[IBIS ver]   4.1
[File name]   sprm642a.ibs
[File Rev]   1.0
[Notes]
   IO cell model for C2000
[Date]   Nov 21, 2013
[Source]   File originated at Texas Instruments
[Copyright]   (c) 2012, Texas Instruments Inc.
[Component]   f771553xptp
[Manufacturer] Texas Instruments
[Package]
| Variable   Typ   Min   Max
R_pkg   0.164   0.00678   0.207
L_pkg   7.99E-09   6.94E-09   9.66E-09
C_pkg   2.73E-12   2.18E-12   3.96E-12
[Pin] signal_name   model_name   R_pin   L_pin   C_pin
1   GPIO10   BCF183350CSHYPBFZ   2.07E-01   9.66E-09   2.25E-12
2   GPIO11   BCF183350CSHYPBFZ   2.03E-01   9.34E-09   3.02E-12
3   VDDSFL1833   NC   1.98E-01   9.27E-09   3.01E-12
4   GPIO12   BCF183350CSHYPBFZ   1.92E-01   8.96E-09   2.97E-12
5   GPIO13   BCF183350CSHYPBFZ   1.90E-01   8.86E-09   2.93E-12
6   GPIO14   BCF183350CSHYPBFZ   1.85E-01   8.70E-09   2.89E-12
7   GPIO15   BCF183350CSHYPBFZ   1.82E-01   8.48E-09   2.84E-12
8   GPIO16   BCF183350CSHYPBFZ   1.79E-01   8.37E-09   2.81E-12
9   GPIO17   BCF183350CSHYPBFZ   1.76E-01   8.17E-09   2.76E-12
10   GPIO18   BCF183350CSHYPBFZ   1.74E-01   8.07E-09   2.70E-12
11   VDDSFL1833   NC   1.73E-01   7.90E-09   2.65E-12
12   GPIO19   BCF183350CSHYPBFZ   1.72E-01   7.79E-09   2.62E-12
13   GPIO20   BCF183350CSHYPBFZ   1.71E-01   7.75E-09   2.59E-12
14   GPIO21   BCF183350CSHYPBFZ   1.71E-01   7.59E-09   2.55E-12
15   VDDSFL   NC   1.72E-01   7.56E-09   2.52E-12
16   VDD   NC   1.72E-01   7.53E-09   2.48E-12
17   VPP   NC   9.16E-02   7.04E-09   2.94E-12
18   GPIO8   BCF3350CSHYPBFZ   1.74E-01   7.41E-09   2.43E-12
19   GPIO9   BCF3350CSHYPBFZ   1.74E-01   7.27E-09   2.40E-12
20   VDDSFL   NC   1.75E-01   7.31E-09   2.44E-12
21   VDD   NC   1.75E-01   7.17E-09   3.56E-12
22   GPIO22   BCF3350CSHYPBFZ   1.77E-01   7.39E-09   2.42E-12
23   GPIO23   BCF3350CSHYPBFZ   1.76E-01   7.29E-09   2.44E-12
24   GPIO24   BCF3350CSHYPBFZ   1.76E-01   7.24E-09   2.41E-12
25   GPIO25   BCF3350CSHYPBFZ   1.75E-01   7.32E-09   2.40E-12
26   VDDSFL   NC   1.75E-01   7.31E-09   2.39E-12
27   GPIO26   BCF3350CSHYPBFZ   1.75E-01   7.38E-09   2.41E-12
28   GPIO27   BCF3350CSHYPBFZ   1.76E-01   7.44E-09   2.40E-12
29   ADCINC4   NC   1.76E-01   7.49E-09   2.43E-12
30   ADCINC3   NC   1.75E-01   7.51E-09   2.50E-12
31   ADCINC2   NC   1.74E-01   7.60E-09   2.55E-12
32   ADCINC1   NC   1.74E-01   7.67E-09   2.60E-12
33   ADCINC0   NC   1.74E-01   7.80E-09   2.65E-12
34   VSSA   NC   1.75E-01   7.84E-09   2.71E-12
35   VREFHI3   NC   9.36E-02   7.64E-09   3.39E-12
36   VDDA   NC   9.37E-02   7.69E-09   3.48E-12
37   VREFHI1   NC   9.43E-02   7.85E-09   3.53E-12
38   ADCINA5   NC   9.49E-02   7.97E-09   3.52E-12
39   ADCINA4   NC   1.80E-01   8.46E-09   2.92E-12
40   ADCINA3   NC   1.82E-01   8.72E-09   2.95E-12
41   ADCINA2   NC   1.86E-01   8.78E-09   2.98E-12
42   ADCINA1   NC   1.90E-01   8.94E-09   3.01E-12
43   ADCINA0   NC   1.95E-01   9.19E-09   3.03E-12
44   ADCINCAL0   NC   2.00E-01   9.52E-09   2.27E-12
45   ADCINCAL1   NC   1.72E-01   9.30E-09   2.25E-12
46   ADCINB0   NC   1.66E-01   9.01E-09   3.05E-12
47   ADCINB1   NC   1.63E-01   8.95E-09   3.04E-12
48   ADCINB2   NC   1.59E-01   8.56E-09   3.00E-12
49   ADCINB3   NC   1.56E-01   8.52E-09   2.95E-12
50   ADCINB4   NC   1.54E-01   8.36E-09   2.90E-12
51   ADCINB5   NC   1.52E-01   8.19E-09   2.84E-12
52   VSSA   NC   8.44E-02   8.01E-09   3.36E-12
53   VREFHI2   NC   8.38E-02   7.79E-09   3.39E-12
54   VDDA   NC   8.35E-02   7.72E-09   3.36E-12
55   VREFHI4   NC   8.31E-02   7.60E-09   3.30E-12
56   ADCIND0   NC   1.53E-01   7.61E-09   2.70E-12
57   ADCIND1   NC   1.52E-01   7.63E-09   2.64E-12
58   ADCIND2   NC   1.52E-01   7.52E-09   2.58E-12
59   ADCIND3   NC   1.52E-01   7.43E-09   2.53E-12
60   ADCIND4   NC   1.53E-01   7.32E-09   2.46E-12
61   VDD   NC   1.58E-01   7.52E-09   2.40E-12
62   VDDSFL   NC   1.57E-01   7.34E-09   2.42E-12
63   GPIO30   BCF3355DSHYPBFZ   1.57E-01   7.16E-09   2.42E-12
64   GPIO28   BCF3385DSHYPBFZ   1.56E-01   7.30E-09   2.41E-12
65   GPIO29   BCF3385DSHYPBFZ   1.55E-01   7.15E-09   2.38E-12
66   GPIO31   BCF3385DSHYPBFZ   1.55E-01   7.23E-09   2.29E-12
67   GPIO32   BCF3385DSHYPBFZ   1.57E-01   7.26E-09   2.32E-12
68   VDDSFL   NC   1.56E-01   7.23E-09   2.41E-12
69   GPIO33   BCF3385DSHYPBFZ   1.53E-01   7.13E-09   2.43E-12
70   GPIO34   BCF3385DSHYPBFZ   1.52E-01   7.18E-09   2.45E-12
71   GPIO35   BCF3385DSHYPBFZ   1.50E-01   7.12E-09   2.45E-12
72   VDD3VFL   NC   7.87E-02   6.94E-09   2.89E-12
73   FLT1   NC   1.46E-01   7.32E-09   2.46E-12
74   FLT2   NC   1.45E-01   7.25E-09   2.48E-12
75   VDDSFL   NC   1.48E-01   7.47E-09   2.58E-12
76   VDD   NC   1.47E-01   7.42E-09   3.55E-12
77   TDI   BCF3335DSHYPBFZ   1.47E-01   7.64E-09   2.64E-12
78   TDO   BCF3335DSHYPBFZ   1.46E-01   7.81E-09   2.67E-12
79   TRSTn   BCF3335CSHYPBFZ   1.46E-01   7.84E-09   2.69E-12
80   TMS   IQ0442FS_40P60P_3X2   1.46E-01   8.01E-09   2.71E-12
81   TCK   IQ0442FS_40P60P_3X2   1.46E-01   8.05E-09   2.75E-12
82   VDDSFL   NC   1.46E-01   8.21E-09   2.79E-12
83   GPIO36   BCF3385DSHYPBFZ   1.46E-01   8.25E-09   2.85E-12
84   GPIO37   BCF3385DSHYPBFZ   1.47E-01   8.41E-09   2.91E-12
85   GPIO38   BCF3385DSHYPBFZ   1.49E-01   8.54E-09   2.96E-12
86   GPIO39   BCF3385DSHYPBFZ   1.52E-01   8.80E-09   2.98E-12
87   GPIO40   BCF3385DSHYPBFZ   1.53E-01   8.92E-09   2.99E-12
88   VDDSFL   NC   1.55E-01   8.99E-09   2.23E-12
89   GPIO41   BCF3385DSHYPBFZ   1.77E-01   9.22E-09   2.18E-12
90   GPIO48   BCF3385DSHYPBFZ   1.73E-01   9.12E-09   2.92E-12
91   VDDSFL   NC   1.69E-01   8.83E-09   2.91E-12
92   ERRORSTS   BCF3350BSHYPBFZ   1.66E-01   8.63E-09   2.87E-12
93   GPIO49   BCF3385DSHYPBFZ   1.63E-01   8.50E-09   2.83E-12
94   GPIO50   BCF3385DSHYPBFZ   1.59E-01   8.25E-09   2.80E-12
95   GPIO51   BCF3385DSHYPBFZ   1.56E-01   8.24E-09   2.75E-12
96   GPIO52   BCF3385DSHYPBFZ   1.52E-01   7.95E-09   2.71E-12
97   GPIO53   BCF3385DSHYPBFZ   1.50E-01   7.79E-09   2.66E-12
98   GPIO54   BCF3385DSHYPBFZ   1.48E-01   7.68E-09   2.61E-12
99   VDDSFL   NC   1.47E-01   7.64E-09   2.57E-12
100   GPIO55   BCF3385DSHYPBFZ   1.47E-01   7.48E-09   2.53E-12
101   GPIO56   BCF3385DSHYPBFZ   1.47E-01   7.31E-09   2.50E-12
102   GPIO57   BCF3385DSHYPBFZ   1.48E-01   7.20E-09   2.46E-12
103   GPIO58   BCF3385DSHYPBFZ   1.48E-01   7.19E-09   2.42E-12
104   GPIO59   BCF3335DSHYPBFZ   1.50E-01   7.14E-09   2.37E-12
105   GPIO60   BCF3385DSHYPBFZ   1.51E-01   6.96E-09   2.34E-12
106   VDDSFL   NC   1.51E-01   7.04E-09   2.33E-12
107   GPIO61   BCF3335DSHYPBFZ   1.52E-01   7.01E-09   2.33E-12
108   GPIO62   BCF3385DSHYPBFZ   1.54E-01   7.06E-09   2.35E-12
109   GPIO63   BCF3385DSHYPBFZ   1.56E-01   7.10E-09   2.35E-12
110   GPIO64   BCF3335DSHYPBFZ   1.59E-01   7.06E-09   2.35E-12
111   GPIO65   BCF3385DSHYPBFZ   1.62E-01   7.29E-09   2.33E-12
112   GPIO66   BCF3335DSHYPBFZ   1.63E-01   7.14E-09   2.38E-12
113   GPIO44   BCF3385DSHYPBFZ   1.65E-01   7.14E-09   2.41E-12
114   VDDSFL   NC   1.66E-01   7.23E-09   2.40E-12
115   GPIO45   BCF3385DSHYPBFZ   1.68E-01   7.30E-09   2.40E-12
116   VDDSFL   NC   1.62E-01   7.25E-09   2.45E-12
117   VDD   NC   1.60E-01   7.30E-09   3.56E-12
118   GPIO133   BCF3350BSHYPBFZ   1.63E-01   7.45E-09   2.52E-12
119   VREGENZ   IQ0440FS_3X2_7LM   1.66E-01   7.60E-09   2.54E-12
120   VDDSFL1   NC   1.69E-01   7.79E-09   2.57E-12
121   X2   NC   1.71E-01   7.78E-09   2.60E-12
122   VSS.OSC   NC   1.74E-01   8.15E-09   2.64E-12
123   X1   NC   1.79E-01   8.15E-09   2.66E-12
124   XRSn   BQ0491FS_3X2_7LM   1.74E-01   8.11E-09   2.71E-12
125   VDDSFL1   NC   1.76E-01   8.29E-09   2.81E-12
126   VDD   NC   6.78E-02   7.88E-09   3.96E-12
127   VDDSFL2   NC   9.38E-02   8.22E-09   3.38E-12
128   GPIO46   GPIOUSBV4_NFS_7LM   1.73E-01   8.62E-09   2.86E-12
129   GPIO47   GPIOUSBV4_NFS_7LM   1.78E-01   8.91E-09   2.91E-12
130   GPIO42   GPIOUSBV4_NFS_7LM   1.83E-01   9.10E-09   2.93E-12
131   GPIO43   GPIOUSBV4_NFS_7LM   1.86E-01   9.13E-09   2.93E-12
132   GPIO67   BCF3385DSHYPBFZ   1.91E-01   9.18E-09   2.19E-12
133   GPIO68   BCF3385DSHYPBFZ   1.84E-01   9.45E-09   2.29E-12
134   GPIO69   BCF3385DSHYPBFZ   1.83E-01   9.11E-09   3.06E-12
135   GPIO70   BCF3335DSHYPBFZ   1.81E-01   9.11E-09   3.04E-12
136   GPIO71   BCF3385DSHYPBFZ   1.80E-01   9.03E-09   3.00E-12
137   VDD   NC   1.79E-01   8.78E-09   2.97E-12
138   VDDSFL   NC   1.77E-01   8.85E-09   2.95E-12
139   GPIO72   BCF3335DSHYPBFZ   1.77E-01   8.55E-09   2.92E-12
140   GPIO73   BCF3385DSHYPBFZ   1.75E-01   8.52E-09   2.88E-12
141   GPIO74   BCF3385DSHYPBFZ   1.74E-01   8.26E-09   2.85E-12
142   GPIO75   BCF3385DSHYPBFZ   1.74E-01   8.18E-09   2.81E-12
143   GPIO76   BCF3385DSHYPBFZ   1.74E-01   8.08E-09   2.77E-12
144   GPIO77   BCF3385DSHYPBFZ   1.74E-01   7.96E-09   2.73E-12
145   GPIO78   BCF3385DSHYPBFZ   1.75E-01   7.90E-09   2.70E-12
146   GPIO79   BCF3385DSHYPBFZ   1.76E-01   7.78E-09   2.66E-12
147   VDDSFL   NC   1.77E-01   7.79E-09   2.63E-12
148   GPIO80   BCF3385DSHYPBFZ   1.78E-01   7.77E-09   2.60E-12
149   GPIO81   BCF3385DSHYPBFZ   1.80E-01   7.75E-09   2.58E-12
150   GPIO82   BCF3385DSHYPBFZ   1.82E-01   7.70E-09   2.55E-12
151   GPIO83   BCF3385DSHYPBFZ   1.85E-01   7.76E-09   2.50E-12
152   VDDSFL   NC   1.81E-01   7.56E-09   2.52E-12
153   VDD   NC   1.82E-01   7.60E-09   3.64E-12
154   GPIO84   BCF3385DSHYPBFZ   1.81E-01   7.62E-09   2.43E-12
155   GPIO85   BCF3385DSHYPBFZ   1.83E-01   7.67E-09   2.46E-12
156   GPIO86   BCF3385DSHYPBFZ   1.83E-01   7.54E-09   2.51E-12
157   GPIO87   BCF3385DSHYPBFZ   1.84E-01   7.64E-09   2.49E-12
158   VDD   NC   1.78E-01   7.56E-09   3.64E-12
159   VDDSFL   NC   1.78E-01   7.62E-09   2.55E-12
160   GPIO0   GPIORETV2_NFS   1.74E-01   7.67E-09   2.55E-12
161   GPIO1   GPIORETV2_NFS   1.74E-01   7.68E-09   2.60E-12
162   GPIO2   GPIORETV2_NFS   1.74E-01   7.66E-09   2.63E-12
163   GPIO3   GPIORETV2_NFS   1.75E-01   7.78E-09   2.67E-12
164   GPIO4   GPIORETV2_NFS   1.76E-01   7.91E-09   2.71E-12
165   GPIO5   GPIORETV2_NFS   1.78E-01   8.06E-09   2.75E-12
166   GPIO6   GPIORETV2_NFS   1.79E-01   8.20E-09   2.78E-12
167   GPIO7   GPIORETV2_NFS   1.82E-01   8.28E-09   2.81E-12
168   VDDSFL   NC   1.84E-01   8.73E-09   2.89E-12
169   VDD   NC   9.91E-02   8.26E-09   3.52E-12
170   GPIO88   BCF3385DSHYPBFZ   1.87E-01   8.74E-09   2.98E-12
171   GPIO89   BCF3385DSHYPBFZ   1.90E-01   8.89E-09   3.03E-12
172   GPIO90   BCF3385DSHYPBFZ   1.94E-01   9.02E-09   3.07E-12
173   GPIO91   BCF3385DSHYPBFZ   1.98E-01   9.32E-09   3.08E-12
174   GPIO92   BCF3385DSHYPBFZ   2.00E-01   9.37E-09   3.09E-12
175   GPIO93   BCF3385DSHYPBFZ   2.02E-01   9.49E-09   3.10E-12
176   GPIO94   BCF3385DSHYPBFZ   2.01E-01   9.61E-09   2.31E-12
| End of package information
|   Component BCF3335DSHYPBFZ
[Component]   BCF3335DSHYPBFZ
[Manufacturer]   Texas Instruments
[Package]
|  variable   typ   min   max
R_pkg   0   0   0
L_pkg   0   0   0
C_pkg   0   0   0
[Pin]   signal_name   model_name   R_pin   L_pin   C_pin
VSS   VSS   GND
VDDS   VDDS   POWER
PAD   PAD   BCF3335DSHYPBFZ
[Model Selector] BCF3335DSHYPBFZ
BCF3335D_WK_PU_ON  Cell operated at 3.3(nom)
|BCF3335D_WK_PU_ON; WEAK_PULLUP_ON
BCF3335D_DRIVER_MODE  Cell operated at 3.3(nom)
|BCF3335D_DRIVER_MODE
BCF3335D_WK_PD_ON  Cell operated at 3.3(nom)
|   Component BCF3385DSHYPBFZ
[Component]   BCF3385DSHYPBFZ
[Manufacturer]   Texas Instruments
[Package]
|  variable   typ   min   max
R_pkg   0   0   0
L_pkg   0   0   0
C_pkg   0   0   0
[Pin]   signal_name   model_name   R_pin   L_pin   C_pin
VSS   VSS   GND
VDDS   VDDS   POWER
PAD   PAD   BCF3385DSHYPBFZ
[Model Selector] BCF3385DSHYPBFZ
BCF3385D_WK_PU_ON  Cell operated at 3.3(nom)
|BCF3385D_WK_PU_ON; WEAK_PULLUP_ON
BCF3385D_DRIVER_MODE  Cell operated at 3.3(nom)
|BCF3385D_DRIVER_MODE
BCF3385D_WK_PD_ON  Cell operated at 3.3(nom)
|   Component BCF183350CSHYPBFZ
[Component]   BCF183350CSHYPBFZ
[Manufacturer]   Texas Instruments
[Package]
|  variable   typ   min   max
R_pkg   0   0   0
L_pkg   0   0   0
C_pkg   0   0   0
[Pin]   signal_name   model_name   R_pin   L_pin   C_pin
VSS   VSS   GND
VDDS   VDDS   POWER
PAD   PAD   BCF183350CSHYPBFZ
[Model Selector] BCF183350CSHYPBFZ
BCF183350C_WK_PU_ON_3P3V  Cell operated at 3.3(nom)
|BCF183350C_WK_PU_ON_3P3V; WEAK_PULLUP_ON
BCF183350C_DRVR_MODE_3P3V  Cell operated at 3.3(nom)
|BCF183350C_DRVR_MODE_3P3V
BCF183350C_WK_PD_ON_3P3V  Cell operated at 3.3(nom)
|BCF183350C_WK_PD_ON_3P3V; WEAK_PULLDOWN_ON
BCF183350C_WK_PU_ON_1P8  Cell operated at 1.8(nom)
|BCF183350C_WK_PU_ON_1P8; WEAK_PULLUP_ON
BCF183350C_DRVR_MODE_1P8  Cell operated at 1.8(nom)
|BCF183350C_DRVR_MODE_1P8
BCF183350C_WK_PD_ON_1P8  Cell operated at 1.8(nom)
|   Component IQ0442FS_40P60P_3X2
[Component]   IQ0442FS_40P60P_3X2
[Manufacturer]   Texas Instruments
[Package]
|  variable   typ   min   max
R_pkg   0   0   0
L_pkg   0   0   0
C_pkg   0   0   0
[Pin]   signal_name   model_name   R_pin   L_pin   C_pin
VSS   VSS   GND
VDDS   VDDS   POWER
PAD   PAD   IQ0442FS_40P60P_3X2
[Model Selector] IQ0442FS_40P60P_3X2
S_40P60P_3X2_7LM_3P3  Cell operated at 3.3(nom)
|IQ0442FS_40P60P_3X2_3P3; PUPD_OFF
0P60P_3X2_7LM_PU_3P3  Cell operated at 3.3(nom)
|IQ0442FS_40P60P_3X2_PU_3P3; PULLUP_ON
0P60P_3X2_7LM_PD_3P3  Cell operated at 3.3(nom)
|   Component IQ0440FS_3X2_7LM
[Component]   IQ0440FS_3X2_7LM
[Manufacturer]   Texas Instruments
[Package]
|  variable   typ   min   max
R_pkg   0   0   0
L_pkg   0   0   0
C_pkg   0   0   0
[Pin]   signal_name   model_name   R_pin   L_pin   C_pin
VSS   VSS   GND
VDDS   VDDS   POWER
PAD   PAD   IQ0440FS_3X2_7LM
[Model Selector] IQ0440FS_3X2_7LM
440FS_3X2_7LM_PD_3P3  Cell operated at 3.3(nom)
|IQ0440FS_3X2_7LM_PD_3P3; PULLDOWN_ON
IQ0440FS_3X2_7LM_3P3  Cell operated at 3.3(nom)
|   Component BQ0491FS_3X2_7LM
[Component]   BQ0491FS_3X2_7LM
[Manufacturer]   Texas Instruments
[Package]
|  variable   typ   min   max
R_pkg   0   0   0
L_pkg   0   0   0
C_pkg   0   0   0
[Pin]   signal_name   model_name   R_pin   L_pin   C_pin
VSS   VSS   GND
VDDS   VDDS   POWER
PAD   PAD   BQ0491FS_3X2_7LM
[Model Selector] BQ0491FS_3X2_7LM
491FS_3X2_7LM_PU_3P3  Cell operated at 3.3(nom)
|BQ0491FS_3X2_7LM_PU_3P3; PULLUP_ON
491FS_3X2_7LM_PZ_3P3  Cell operated at 3.3(nom)
|   Component GPIORETV2_NFS
[Component]   GPIORETV2_NFS
[Manufacturer]   Texas Instruments
[Package]
|  variable   typ   min   max
R_pkg   0   0   0
L_pkg   0   0   0
C_pkg   0   0   0
[Pin]   signal_name   model_name   R_pin   L_pin   C_pin
VSS   VSS   GND
VDDS   VDDS   POWER
PAD   PAD   GPIORETV2_NFS
[Model Selector] GPIORETV2_NFS
GPIORET_WK_PD_ON_3P3  Cell operated at 3.3(nom)
|GPIORET_WK_PD_ON_3P3; WEAK_PULLDOWN_ON
RET_8MA_OPEN_DRAIN  Cell operated at 3.3(nom)
|RET_8MA_OPEN_DRAIN; 8MA_OPEN_DRAIN_SLW
RET_DRVR_2MA_PUPDOFF  Cell operated at 3.3(nom)
|RET_DRVR_2MA_PUPDOFF
RET_4MA_OPEN_DRAIN  Cell operated at 3.3(nom)
|RET_4MA_OPEN_DRAIN; 4MA_OPEN_DRAIN
GPIORET_WK_PU_ON_3P3  Cell operated at 3.3(nom)
|GPIORET_WK_PU_ON_3P3; WEAK_PULLUP_ON
RET_2MA_OPEN_DRAIN  Cell operated at 3.3(nom)
|RET_2MA_OPEN_DRAIN; 2MA_OPEN_DRAIN
RET_DRVR_8MA_PUPDOFF  Cell operated at 3.3(nom)
|RET_DRVR_8MA_PUPDOFF
RET_DRVR_MODE_8MA_PUPDOFF_SLEW  Cell operated at 3.3(nom)
|RET_DRVR_MODE_8MA_PUPDOFF_SLEW
RET_DRVR_MODE_4MA_PUPDOFF  Cell operated at 3.3(nom)
|RET_DRVR_MODE_4MA_PUPDOFF
RET_8MA_OPEN_DRAIN_3P3  Cell operated at 3.3(nom)
|   Component BCF3335CSHYPBFZ
[Component]   BCF3335CSHYPBFZ
[Manufacturer]   Texas Instruments
[Package]
|  variable   typ   min   max
R_pkg   0   0   0
L_pkg   0   0   0
C_pkg   0   0   0
[Pin]   signal_name   model_name   R_pin   L_pin   C_pin
VSS   VSS   GND
VDDS   VDDS   POWER
PAD   PAD   BCF3335CSHYPBFZ
[Model Selector] BCF3335CSHYPBFZ
BCF3335C_WK_PU_ON_3P3  Cell operated at 3.3(nom)
|BCF3335C_WK_PU_ON_3P3; WEAK_PULLUP_ON
BCF3335C_DRIVER_MODE_3P3  Cell operated at 3.3(nom)
|BCF3335C_DRIVER_MODE_3P3
BCF3335C_WK_PD_ON_3P3  Cell operated at 3.3(nom)
|   Component BCF3350CSHYPBFZ
[Component]   BCF3350CSHYPBFZ
[Manufacturer]   Texas Instruments
[Package]
|  variable   typ   min   max
R_pkg   0   0   0
L_pkg   0   0   0
C_pkg   0   0   0
[Pin]   signal_name   model_name   R_pin   L_pin   C_pin
VSS   VSS   GND
VDDS   VDDS   POWER
PAD   PAD   BCF3350CSHYPBFZ
[Model Selector] BCF3350CSHYPBFZ
BCF3350C_WK_PU_ON_3P3  Cell operated at 3.3(nom)
|BCF3350C_WK_PU_ON_3P3; WEAK_PULLUP_ON
BCF3350C_DRIVER_MODE_3P3  Cell operated at 3.3(nom)
|BCF3350C_DRIVER_MODE_3P3
BCF3350C_WK_PD_ON_3P3  Cell operated at 3.3(nom)
|   Component BCF3350BSHYPBFZ
[Component]   BCF3350BSHYPBFZ
[Manufacturer]   Texas Instruments
[Package]
|  variable   typ   min   max
R_pkg   0   0   0
L_pkg   0   0   0
C_pkg   0   0   0
[Pin]   signal_name   model_name   R_pin   L_pin   C_pin
VSS   VSS   GND
VDDS   VDDS   POWER
PAD   PAD   BCF3350BSHYPBFZ
[Model Selector] BCF3350BSHYPBFZ
BCF3350B_WK_PU_ON_3P3  Cell operated at 3.3(nom)
|BCF3350B_WK_PU_ON_3P3; WEAK_PULLUP_ON
BCF3350B_DRIVER_MODE_3P3  Cell operated at 3.3(nom)
|BCF3350B_DRIVER_MODE_3P3
BCF3350B_WK_PD_ON_3P3  Cell operated at 3.3(nom)
|   Component GPIOUSBV4_NFS_7LM
[Component]   GPIOUSBV4_NFS_7LM
[Manufacturer]   Texas Instruments
[Package]
|  variable   typ   min   max
R_pkg   0   0   0
L_pkg   0   0   0
C_pkg   0   0   0
[Pin]   signal_name   model_name   R_pin   L_pin   C_pin
VSS   VSS   GND
VDDS   VDDS   POWER
PAD   PAD   GPIOUSBV4_NFS_7LM
[Model Selector] GPIOUSBV4_NFS_7LM
GPIOUSB_WK_PD_ON_3P3  Cell operated at 3.3(nom)
|GPIOUSB_WK_PD_ON_3P3; WEAK_PULLDOWN_ON
USB_8MA_OPEN_DRAIN_SLW  Cell operated at 3.3(nom)
|USB_8MA_OPEN_DRAIN_SLW; 8MA_OPEN_DRAIN_SLW
USB_DRVR_2MA_PUPDOFF  Cell operated at 3.3(nom)
|USB_DRVR_2MA_PUPDOFF
USB_4MA_OPEN_DRAIN  Cell operated at 3.3(nom)
|USB_4MA_OPEN_DRAIN; 4MA_OPEN_DRAIN
GPIOUSB_WK_PU_ON_3P3  Cell operated at 3.3(nom)
|GPIOUSB_WK_PU_ON_3P3; WEAK_PULLUP_ON
USB_2MA_OPEN_DRAIN  Cell operated at 3.3(nom)
|USB_2MA_OPEN_DRAIN; 2MA_OPEN_DRAIN
USB_DRVR_8MA_PUPDOFF  Cell operated at 3.3(nom)
|USB_DRVR_8MA_PUPDOFF
USB_DRVR_8MA_PUPDOFF_SLW  Cell operated at 3.3(nom)
|USB_DRVR_8MA_PUPDOFF_SLW
USB_DRVR_4MA_PUPDOFF  Cell operated at 3.3(nom)
|USB_DRVR_4MA_PUPDOFF
USB_8MA_OPEN_DRAIN  Cell operated at 3.3(nom)
|   Component BCF3355DSHYPBFZ
[Component]   BCF3355DSHYPBFZ
[Manufacturer]   Texas Instruments
[Package]
|  variable   typ   min   max
R_pkg   0   0   0
L_pkg   0   0   0
C_pkg   0   0   0
[Pin]   signal_name   model_name   R_pin   L_pin   C_pin
VSS   VSS   GND
VDDS   VDDS   POWER
PAD   PAD   BCF3355DSHYPBFZ
[Model Selector] BCF3355DSHYPBFZ
BCF3355D_WK_PU_ON_3P3  Cell operated at 3.3(nom)
|BCF3355D_WK_PU_ON_3P3; WEAK_PULLUP_ON
BCF3355D_DRIVER_MODE_3P3  Cell operated at 3.3(nom)
|BCF3355D_DRIVER_MODE_3P3
BCF3355D_WK_PD_ON_3P3  Cell operated at 3.3(nom)
| Models and submodels in the file (51): BCF3335D_WK_PU_ON (Input), BCF3335D_DRIVER_MODE (I/O), BCF3335D_WK_PD_ON (Input), BCF3385D_WK_PU_ON (Input), BCF3385D_DRIVER_MODE (I/O), BCF3385D_WK_PD_ON (Input), BCF183350C_WK_PU_ON_1P8 (Input), BCF183350C_DRVR_MODE_1P8 (I/O), BCF183350C_WK_PD_ON_1P8 (Input), BCF183350C_WK_PU_ON_3P3V (Input), BCF183350C_DRVR_MODE_3P3V (I/O), BCF183350C_WK_PD_ON_3P3V (Input), S_40P60P_3X2_7LM_3P3 (Input), 0P60P_3X2_7LM_PU_3P3 (Input), 0P60P_3X2_7LM_PD_3P3 (Input), 440FS_3X2_7LM_PD_3P3 (Input), IQ0440FS_3X2_7LM_3P3 (Input), 491FS_3X2_7LM_PU_3P3 (I/O), 491FS_3X2_7LM_PZ_3P3 (I/O), GPIORET_WK_PD_ON_3P3 (Input), RET_8MA_OPEN_DRAIN (I/O_open_drain), RET_DRVR_2MA_PUPDOFF (I/O), RET_4MA_OPEN_DRAIN (I/O_open_drain), GPIORET_WK_PU_ON_3P3 (Input), RET_2MA_OPEN_DRAIN (I/O_open_drain), RET_DRVR_8MA_PUPDOFF (I/O), RET_DRVR_MODE_8MA_PUPDOFF_SLEW (I/O), RET_DRVR_MODE_4MA_PUPDOFF (I/O), RET_8MA_OPEN_DRAIN_3P3 (I/O_open_drain), BCF3335C_WK_PU_ON_3P3 (Input), BCF3335C_DRIVER_MODE_3P3 (I/O), BCF3335C_WK_PD_ON_3P3 (Input), BCF3350C_WK_PU_ON_3P3 (Input), BCF3350C_DRIVER_MODE_3P3 (I/O), BCF3350C_WK_PD_ON_3P3 (Input), BCF3350B_WK_PU_ON_3P3 (Input), BCF3350B_DRIVER_MODE_3P3 (I/O), BCF3350B_WK_PD_ON_3P3 (Input), GPIOUSB_WK_PD_ON_3P3 (Input), USB_8MA_OPEN_DRAIN_SLW (I/O_open_drain), USB_DRVR_2MA_PUPDOFF (I/O), USB_4MA_OPEN_DRAIN (I/O_open_drain), GPIOUSB_WK_PU_ON_3P3 (Input), USB_2MA_OPEN_DRAIN (I/O_open_drain), USB_DRVR_8MA_PUPDOFF (I/O), USB_DRVR_8MA_PUPDOFF_SLW (I/O), USB_DRVR_4MA_PUPDOFF (I/O), USB_8MA_OPEN_DRAIN (I/O_open_drain), BCF3355D_WK_PU_ON_3P3 (Input), BCF3355D_DRIVER_MODE_3P3 (I/O), BCF3355D_WK_PD_ON_3P3 (Input)
